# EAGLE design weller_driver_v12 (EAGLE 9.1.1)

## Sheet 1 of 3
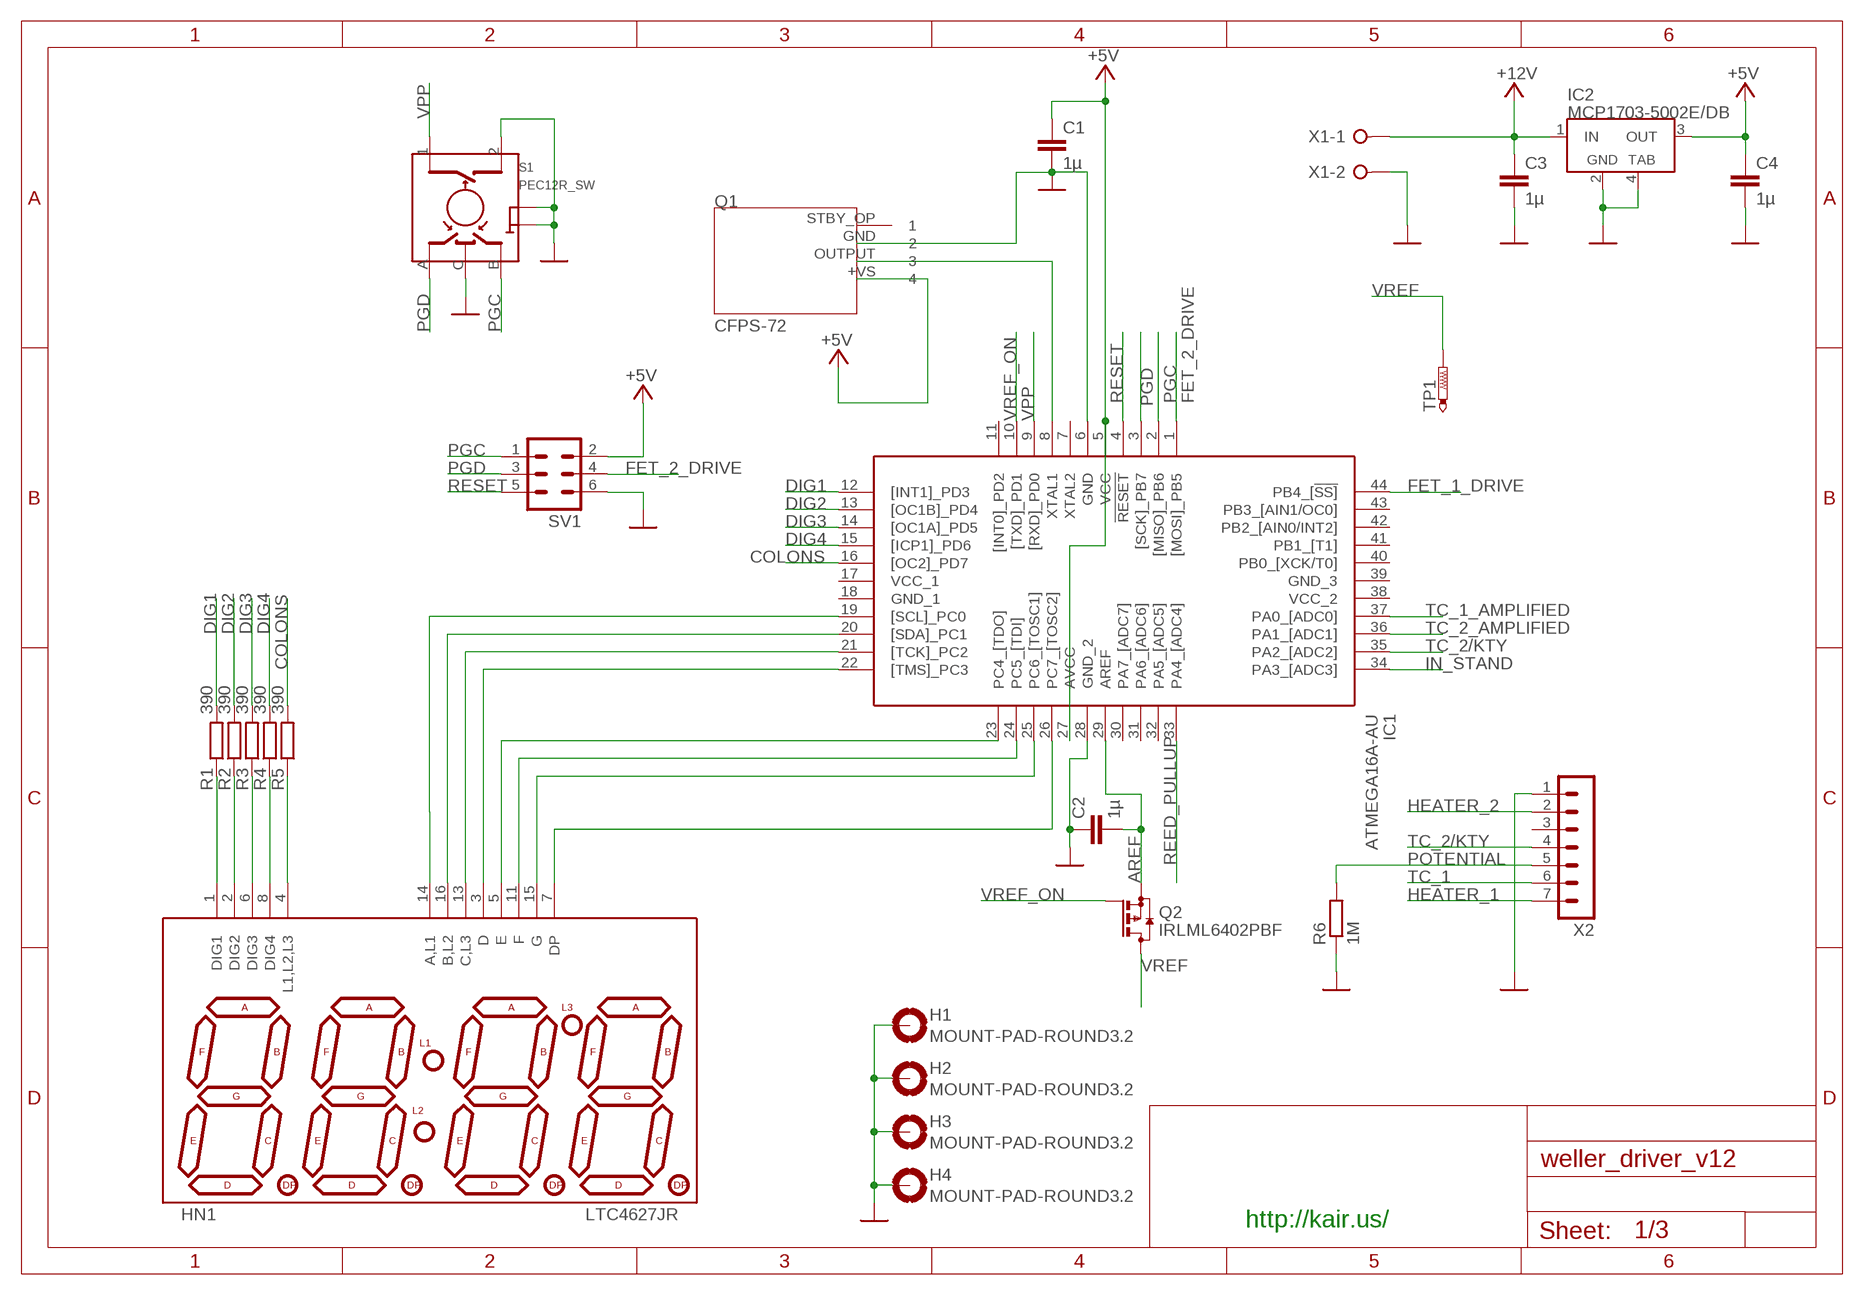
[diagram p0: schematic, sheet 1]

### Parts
C1  1µ  C-EUC0805  [C0805]
C2  1µ  C-EUC0805  [C0805]
C3  1µ  C-EUC0805  [C0805]
C4  1µ  C-EUC0805  [C0805]
H1  MOUNT-PAD-ROUND3.2  [3,2-PAD]
H2  MOUNT-PAD-ROUND3.2  [3,2-PAD]
H3  MOUNT-PAD-ROUND3.2  [3,2-PAD]
H4  MOUNT-PAD-ROUND3.2  [3,2-PAD]
HN1  LTC4627JR  [7-SEGMENT-4DIGIT-YOUNGSUN]
IC1  ATMEGA16A-AU  [ATMEGA16A-AU]
IC2  MCP1703-5002E/DB  VREG_3PIN_FIXED_TAB-SOT223  [SOT223]
Q1  CFPS-72  [CFPS-72]
Q2  IRLML6402PBF  [IRML6402PBF]
R1  390  R-EU_R0805  [R0805]
R2  390  R-EU_R0805  [R0805]
R3  390  R-EU_R0805  [R0805]
R4  390  R-EU_R0805  [R0805]
R5  390  R-EU_R0805  [R0805]
R6  1M  R-EU_R0805  [R0805]
S1  PEC12R_SW  [ALPS_EC12E_SW]
SV1  MA03-2  [MA03-2]
TP1  PTR1PAD1-13  [P1-13]
X1  W237-02P  [W237-132]
X2  MA07-1  [MA07-1]

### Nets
+5V [supply]: C1.1 C4.1 IC1.5(VCC) IC1.27(AVCC) IC2.3(OUT) Q1.+VS SV1.2 ; also sheet 2
+12V [iron_power]: C3.1 IC2.1(IN) X1.1 ; also sheet 2
AREF: C2.2 IC1.29(AREF) Q2.2(S)
COLONS: IC1.16([OC2]_PD7) R5.2
DIG1: IC1.12([INT1]_PD3) R1.2
DIG2: IC1.13([OC1B]_PD4) R2.2
DIG3: IC1.14([OC1A]_PD5) R3.2
DIG4: IC1.15([ICP1]_PD6) R4.2
FET_1_DRIVE: IC1.44(PB4_[!SS]) ; also sheet 2
FET_2_DRIVE: IC1.1([MOSI]_PB5) SV1.4 ; also sheet 2
GND [supply]: C1.2 C2.1 C3.2 C4.2 H1.B3,2(MOUNT) H2.B3,2(MOUNT) H3.B3,2(MOUNT) H4.B3,2(MOUNT) IC1.6(GND) IC1.28(GND_2) IC2.2(GND) IC2.4(GND1) Q1.GND R6.1 S1.2 S1.C S1.GND1(GND) S1.GND2(GND) SV1.6 X1.2 X2.1 ; also sheet 2
HEATER_1 [iron_power]: X2.7 ; also sheet 2
HEATER_2 [iron_power]: X2.2 ; also sheet 2
IN_STAND: IC1.34(PA3_[ADC3]) ; also sheet 2
N$1: HN1.1(DIG1) R1.1
N$2: HN1.2(DIG2) R2.1
N$3: HN1.6(DIG3) R3.1
N$4: HN1.8(DIG4) R4.1
N$7: HN1.5(E) IC1.23(PC4_[TDO])
N$8: IC1.8(XTAL1) Q1.OUTPUT
N$9: HN1.14(A,L1) IC1.19([SCL]_PC0)
N$10: HN1.4(L1,L2,L3) R5.1
N$11: HN1.13(C,L3) IC1.21([TCK]_PC2)
N$13: HN1.16(B,L2) IC1.20([SDA]_PC1)
N$14: HN1.3(D) IC1.22([TMS]_PC3)
N$15: HN1.11(F) IC1.24(PC5_[TDI])
N$16: HN1.15(G) IC1.25(PC6_[TOSC1])
N$17: HN1.7(DP) IC1.26(PC7_[TOSC2])
PGC: IC1.2([MISO]_PB6) S1.B SV1.1
PGD: IC1.3([SCK]_PB7) S1.A SV1.3
POTENTIAL: R6.2 X2.5
REED_PULLUP: IC1.33(PA4_[ADC4]) ; also sheet 2
RESET: IC1.4(!RESET) SV1.5
TC_1: X2.6 ; also sheet 2
TC_1_AMPLIFIED: IC1.37(PA0_[ADC0]) ; also sheet 2
TC_2/KTY: IC1.35(PA2_[ADC2]) X2.4 ; also sheet 2
TC_2_AMPLIFIED: IC1.36(PA1_[ADC1]) ; also sheet 2
VPP: IC1.9([RXD]_PD0) S1.1
VREF: Q2.3(D) TP1.TP ; also sheet 2
VREF_ON: IC1.10([TXD]_PD1) Q2.1(G)
Unconnected: IC1.7(XTAL2) IC1.11([INT0]_PD2) IC1.30(PA7_[ADC7]) IC1.31(PA6_[ADC6]) IC1.32(PA5_[ADC5]) IC1.40(PB0_[XCK/T0]) IC1.41(PB1_[T1]) IC1.42(PB2_[AIN0/INT2]) IC1.43(PB3_[AIN1/OC0]) Q1.STBY_OP X2.3

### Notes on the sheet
- http://kair.us/

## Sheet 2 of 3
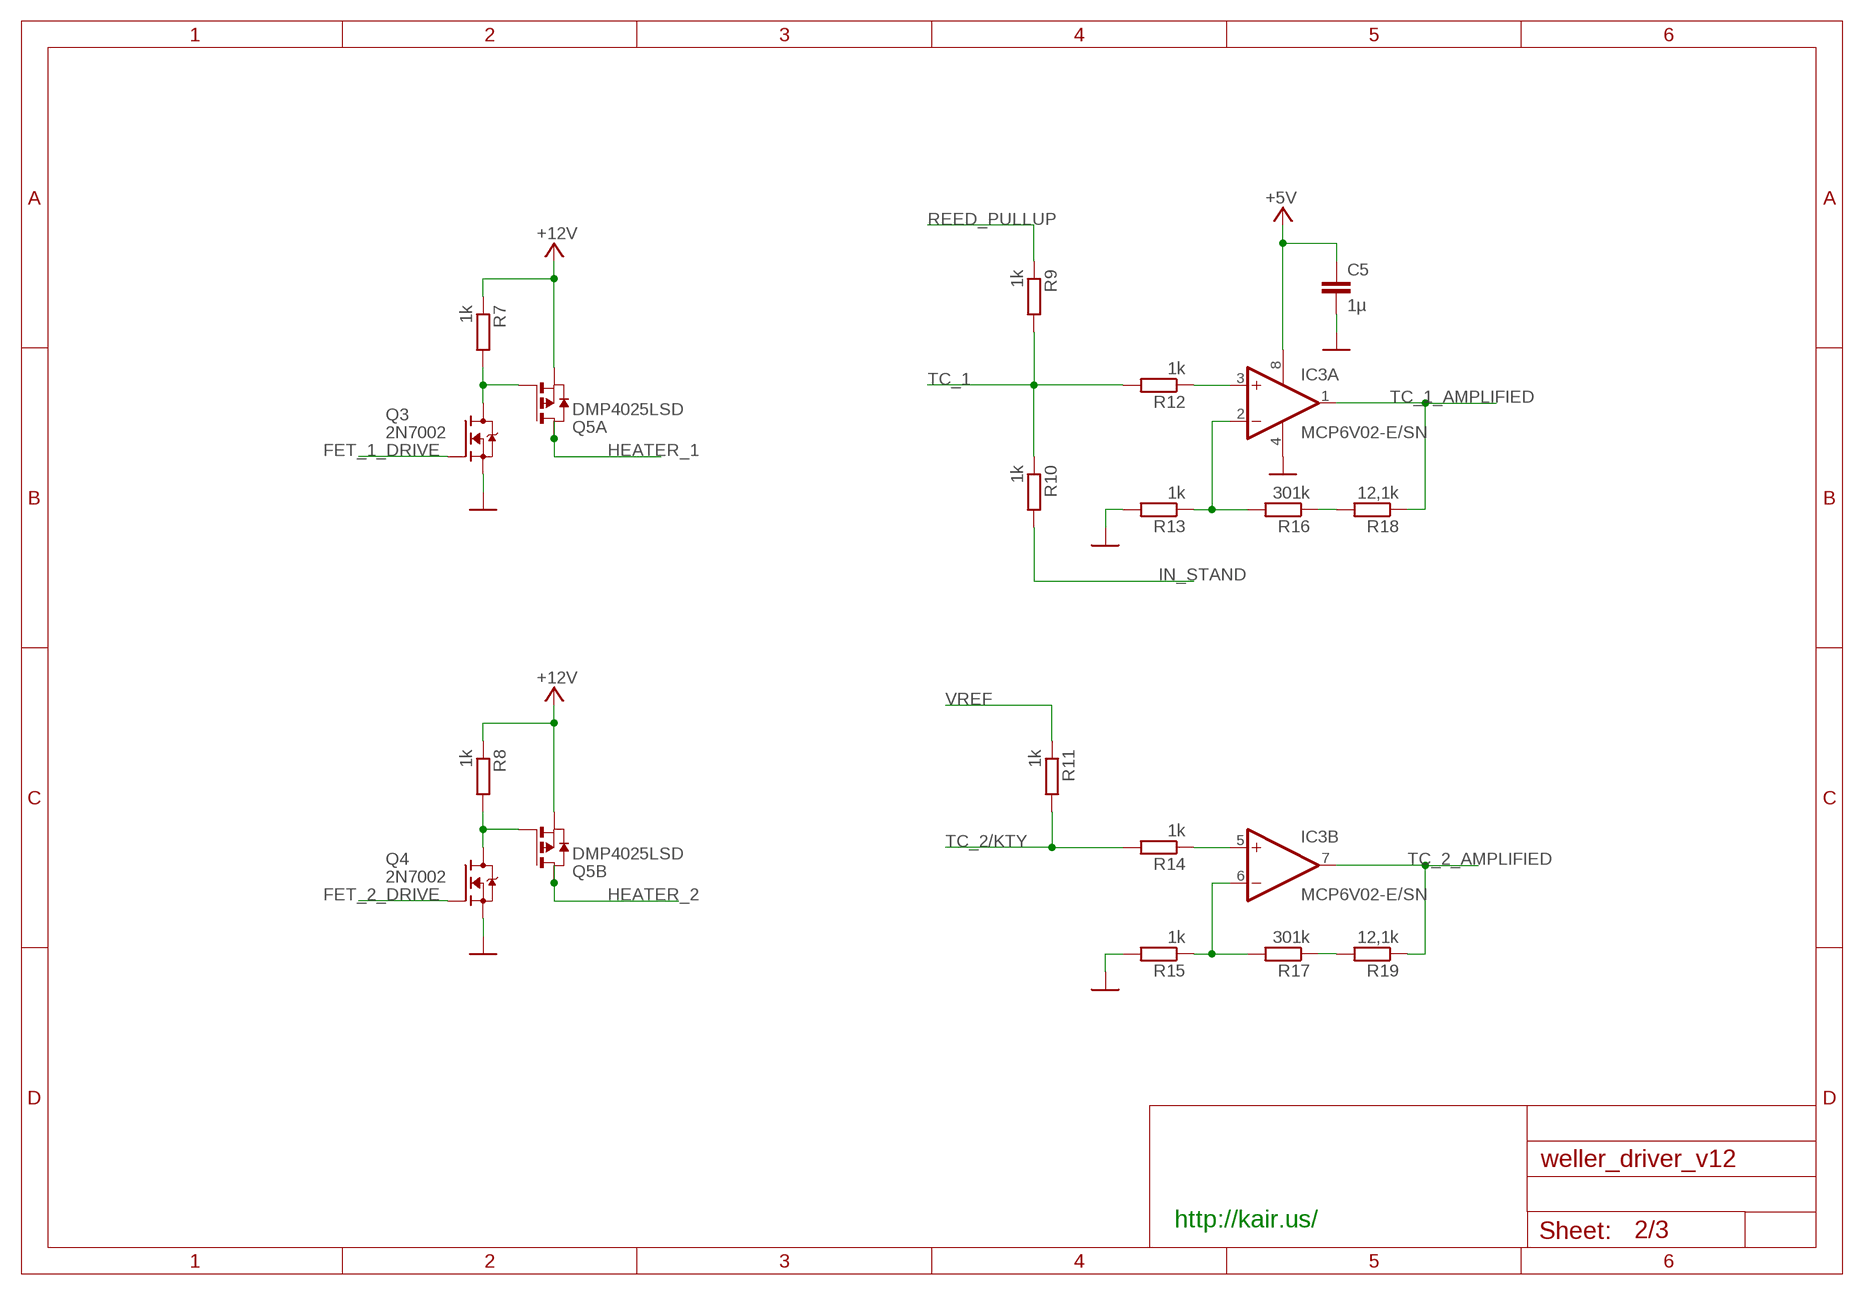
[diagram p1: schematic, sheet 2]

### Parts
C5  1µ  C-EUC0805  [C0805]
IC3  MCP6V02-E/SN  MCP602SN  [SO08]
Q3  2N7002  TRANSISTOR_FET_BS170-SOT-23  [SOT-23]
Q4  2N7002  TRANSISTOR_FET_BS170-SOT-23  [SOT-23]
Q5  DMP4025LSD  PMOS2SO8  [SO08]
R7  1k  R-EU_R0805  [R0805]
R8  1k  R-EU_R0805  [R0805]
R9  1k  R-EU_R0805  [R0805]
R10  1k  R-EU_R0805  [R0805]
R11  1k  R-EU_R0805  [R0805]
R12  1k  R-EU_R0805  [R0805]
R13  1k  R-EU_R0805  [R0805]
R14  1k  R-EU_R0805  [R0805]
R15  1k  R-EU_R0805  [R0805]
R16  301k  R-EU_R0805  [R0805]
R17  301k  R-EU_R0805  [R0805]
R18  12,1k  R-EU_R0805  [R0805]
R19  12,1k  R-EU_R0805  [R0805]

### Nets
+5V [supply]: C5.1 IC3.8(P:V+) ; also sheet 1
+12V [iron_power]: Q5.1(A:S) Q5.3(B:S) R7.1 R8.1 ; also sheet 1
FET_1_DRIVE: Q3.1(G) ; also sheet 1
FET_2_DRIVE: Q4.1(G) ; also sheet 1
GND [supply]: C5.2 IC3.4(P:V-) Q3.2(S) Q4.2(S) R13.2 R15.2 ; also sheet 1
HEATER_1 [iron_power]: Q5.7(A:D) Q5.8(A:D2) ; also sheet 1
HEATER_2 [iron_power]: Q5.5(B:D2) Q5.6(B:D) ; also sheet 1
IN_STAND: R10.2 ; also sheet 1
N$5: R16.1 R18.2
N$6: R17.1 R19.2
N$22: IC3.3(A:+IN) R12.1
N$23: IC3.2(A:-IN) R13.1 R16.2
N$25: IC3.6(B:-IN) R15.1 R17.2
N$27: IC3.5(B:+IN) R14.1
N$28: Q3.3(D) Q5.2(A:G) R7.2
N$42: Q4.3(D) Q5.4(B:G) R8.2
REED_PULLUP: R9.1 ; also sheet 1
TC_1: R9.2 R10.1 R12.2 ; also sheet 1
TC_1_AMPLIFIED: IC3.1(A:OUT) R18.1 ; also sheet 1
TC_2/KTY: R11.2 R14.2 ; also sheet 1
TC_2_AMPLIFIED: IC3.7(B:OUT) R19.1 ; also sheet 1
VREF: R11.1 ; also sheet 1

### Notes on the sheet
- http://kair.us/

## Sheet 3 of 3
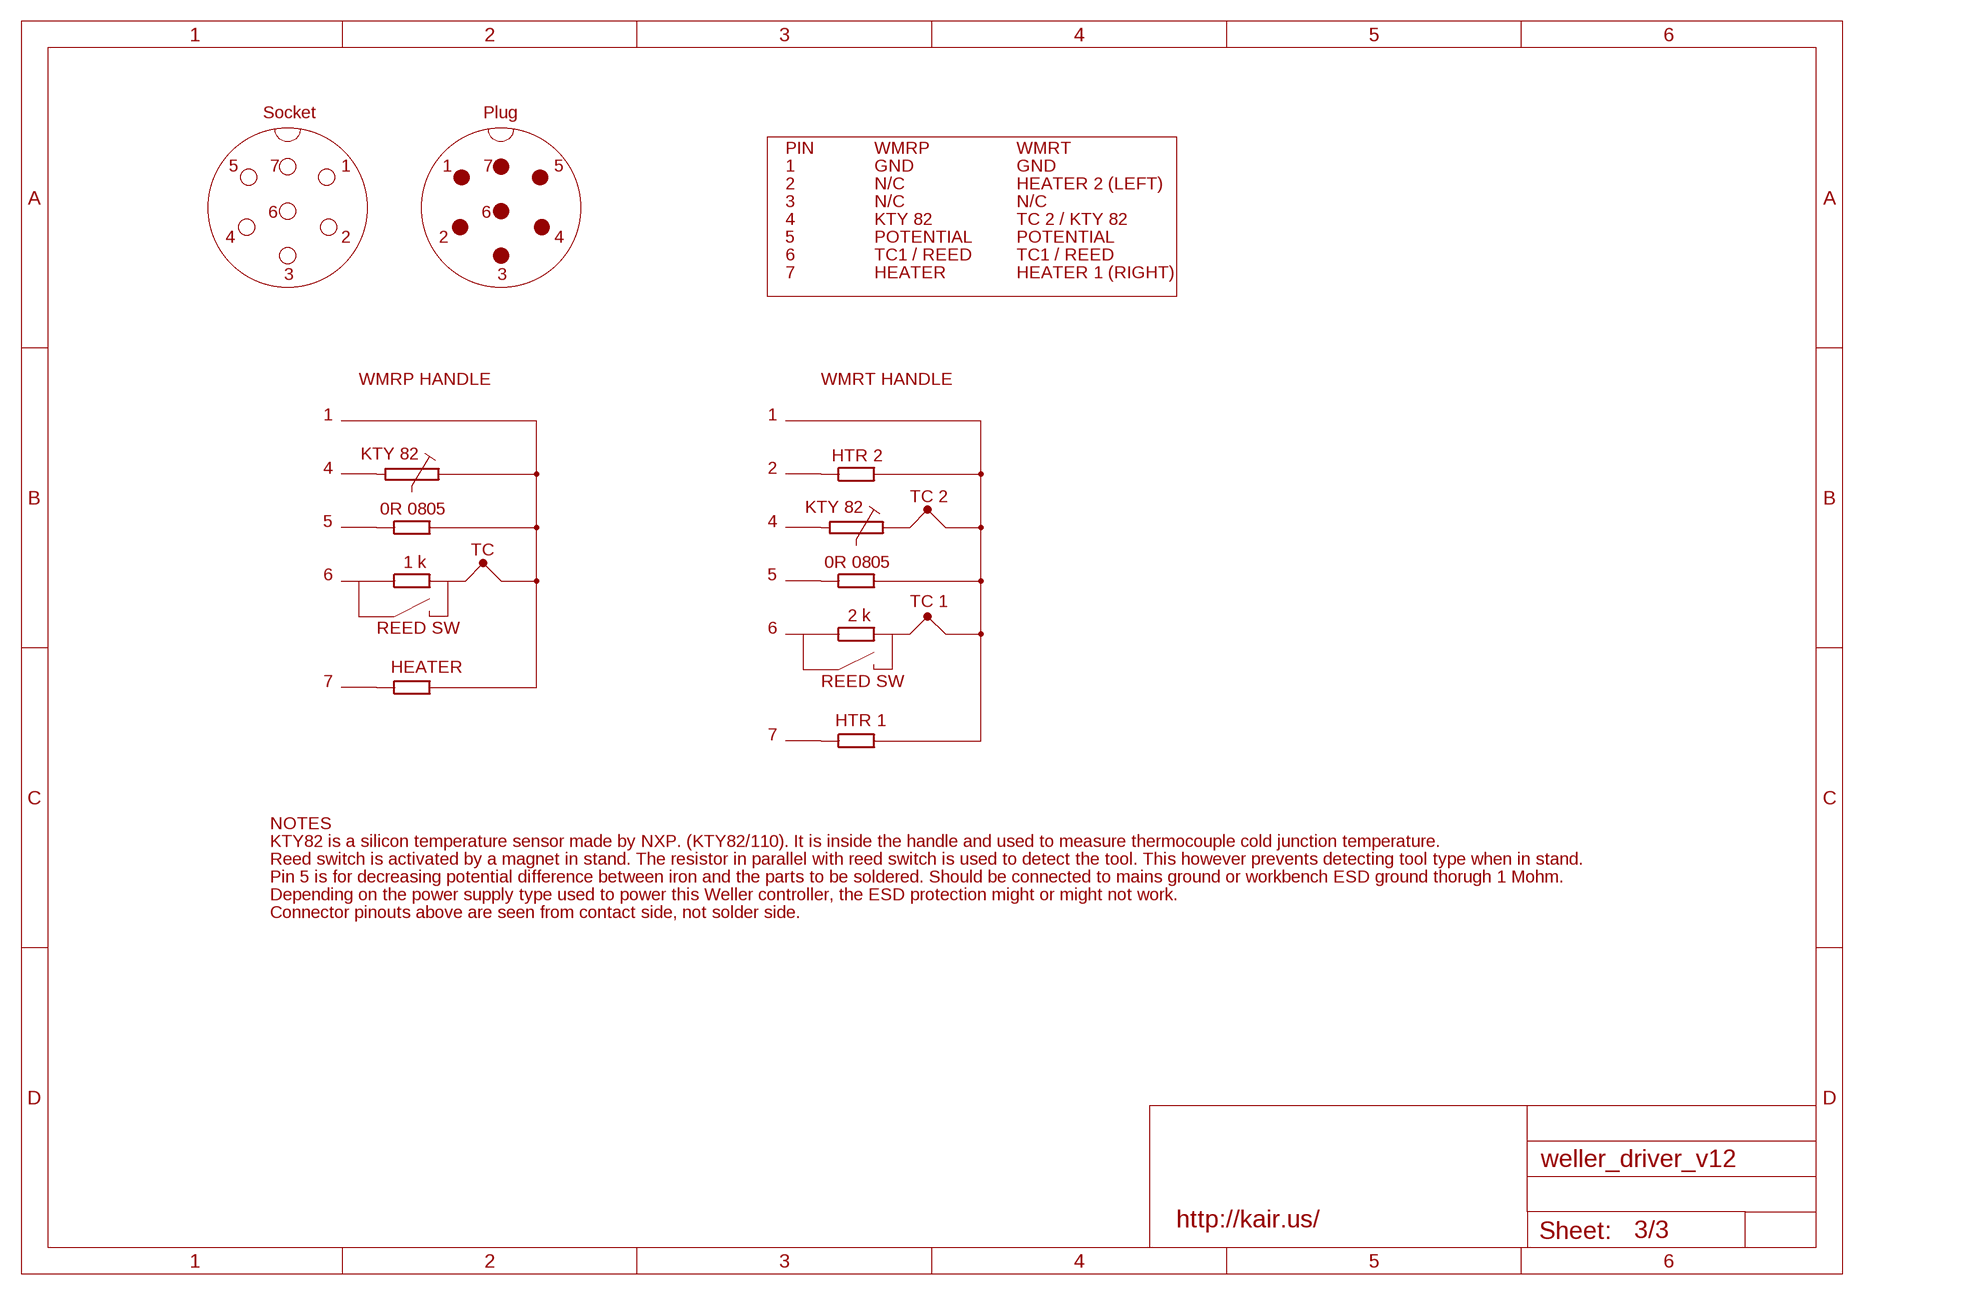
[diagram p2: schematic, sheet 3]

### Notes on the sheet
- Socket | Plug
- PIN | WMRP | WMRT
- 5 | 7 | 1 | 1 | 7 | 5 | 1 | GND | GND
- 2 | N/C | HEATER 2 (LEFT)
- 3 | N/C | N/C
- 6 | 6
- 4 | KTY 82 | TC 2 / KTY 82
- 4 | 2 | 2 | 4 | 5 | POTENTIAL | POTENTIAL
- 6 | TC1 / REED | TC1 / REED
- 3 | 3 | 7 | HEATER | HEATER 1 (RIGHT)
- WMRP HANDLE | WMRT HANDLE
- 1 | 1
- KTY 82 | HTR 2
- 4 | 2
- TC 2
- 0R 0805 | KTY 82
- 5 | 4
- TC
- 1 k | 0R 0805
- 6 | 5
- TC 1
- 2 k
- REED SW | 6
- HEATER
- 7 | REED SW
- HTR 1
- 7
- NOTES
- KTY82 is a silicon temperature sensor made by NXP. (KTY82/110). It is inside the handle and used to measure thermocouple cold junction temperature.
- Reed switch is activated by a magnet in stand. The resistor in parallel with reed switch is used to detect the tool. This however prevents detecting tool type when in stand.
- Pin 5 is for decreasing potential difference between iron and the parts to be soldered. Should be connected to mains ground or workbench ESD ground thorugh 1 Mohm.
- Depending on the power supply type used to power this Weller controller, the ESD protection might or might not work.
- Connector pinouts above are seen from contact side, not solder side.
- http://kair.us/

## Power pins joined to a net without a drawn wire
GND_1: IC1.18(GND_1)
GND_3: IC1.39(GND_3)
VCC_1: IC1.17(VCC_1)
VCC_2: IC1.38(VCC_2)

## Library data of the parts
C1-C5 = dual_atari:C-EU: CAPACITOR, European symbol
H1-H4 = dual_atari:MOUNT-PAD-ROUND: MOUNTING PAD, round
HN1 = omat:LTC4627JR: This is a part for the 4-Digit 7-segment LEDs from Young Sun. Different from the Digikey LEDs, all 16 pins are used. The LONGPADS Variant is used for a test jig, but you may like it because there is more pad to solder to. If you are concerned about routing space, the standard works just fine though.
IC1 = SamacSys_Parts:ATMEGA16A-AU: ATMEGA16A-AU, 8 bit AVR Microcontroller 16MHz 16, 512kB, B Flash, 1kb RAM, I2C SPI 44-Pin TQFP Source: Datasheet; DESCRIPTION: ATMEGA16A-AU, 8 bit AVR Microcontroller 16MHz 16, 512kB, B Flash, 1kb RAM, I2C SPI 44-Pin TQFP; HEIGHT: 1.2mm; MANUFACTURER_NAME: Microchip; MANUFACTURER_PART_NUMBER: ATMEGA16A-AU; MOUSER_PART_NUMBER: 556-ATMEGA16A-AU; MOUSER_PRICE-STOCK: https://www.mouser.com/Search/Refine.aspx?Keyword=556-ATMEGA16A-AU
IC2 = omat:VREG_3PIN_FIXED_TAB
IC3 = omat:MCP602: Single Op Amp 2.7V to 6.0V Single Supply CMOS Source: http://ww1.microchip.com/downloads/en/DeviceDoc/21314g.pdf
Q1 = CFPS-72:CFPS-72
Q2 = IRLML6402PBF:IRLML6402PBF: P-CHANNEL MOS FET
Q3 Q4 = omat:TRANSISTOR_FET_BS170: N-Channel Enhancement Mode Field Effect Transistor
Q5 = omat:PMOS2: DUAL 30V P-CHANNEL ENHANCEMENT MODE MOSFET Source: Data sheet SOP8 Source: Data sheet MSOP8
R1-R19 = dual_atari:R-EU_: RESISTOR, European symbol
S1 = omat:PEC12R_SW
SV1 = con-lstb:MA03-2: PIN HEADER; OC_FARNELL: unknown; OC_NEWARK: unknown
TP1 = testpad:PTR1: TEST PIN
X1 = omat:W237-02P: WAGO SREW CLAMP; OC_FARNELL: unknown; OC_NEWARK: unknown
X2 = omat:MA07-1: PIN HEADER; OC_FARNELL: unknown; OC_NEWARK: unknown

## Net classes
1 supply: width 0.4 mm, drill 0.7 mm, clearance 0.25 mm
2 iron_power: width 1 mm, drill 0.7 mm, clearance 0.25 mm

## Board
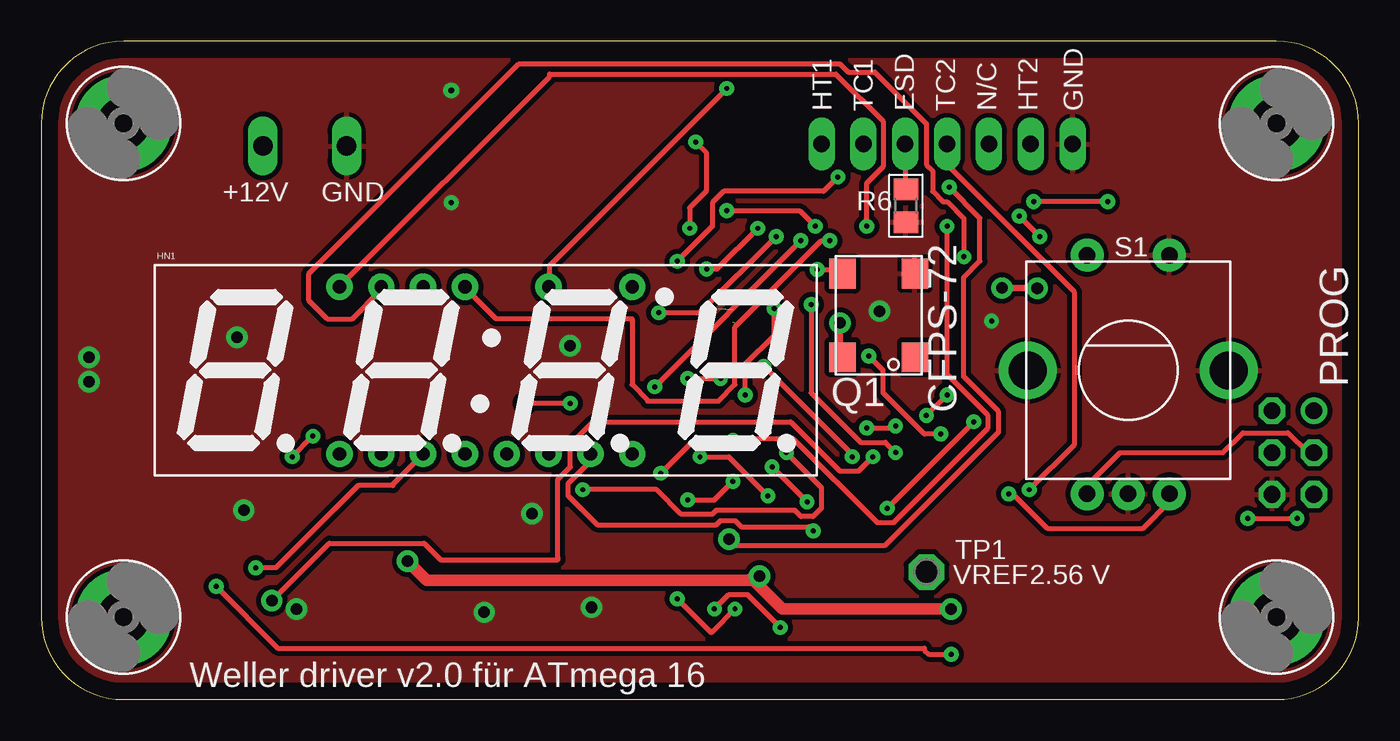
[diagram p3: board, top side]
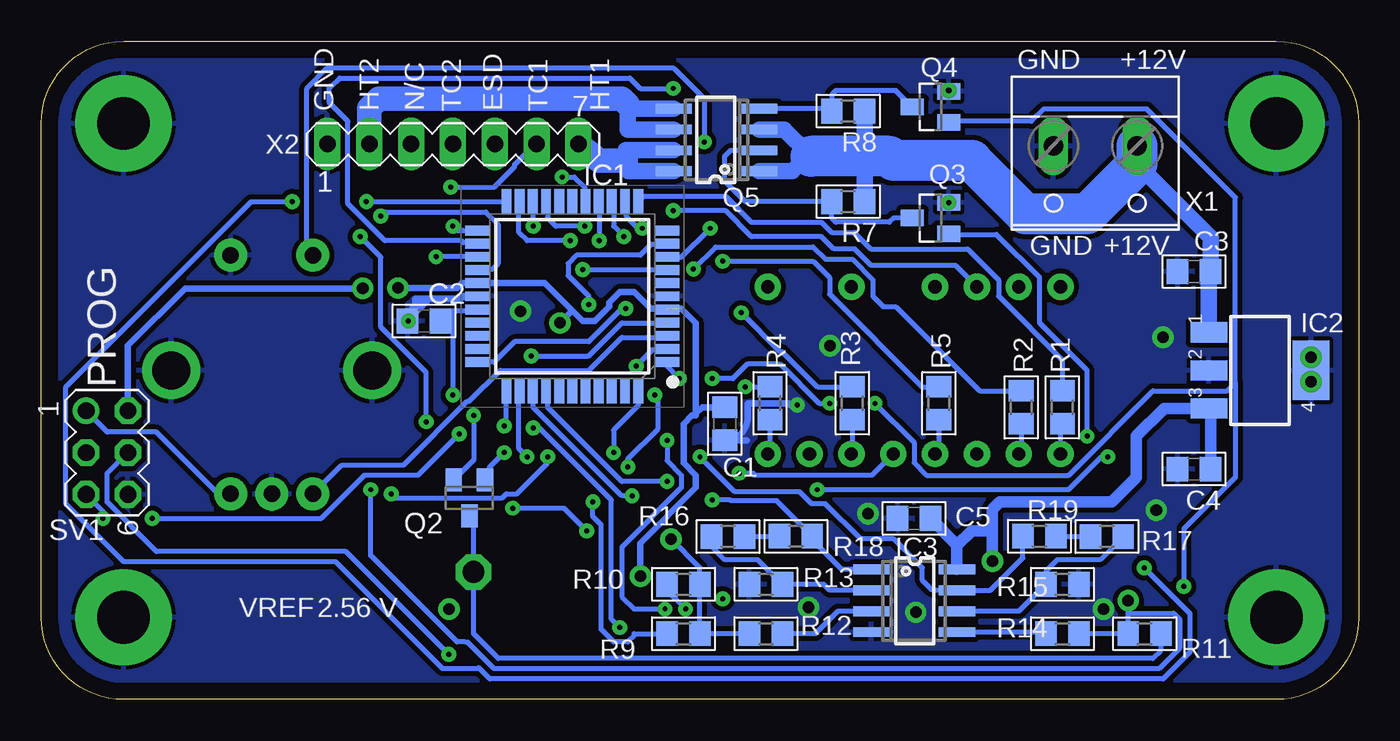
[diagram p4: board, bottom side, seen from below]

Size 80 x 40 mm. Coordinates in mm from the lower left corner, seen from the top.
Outline: 75,0 arc90 80,5 80,35 arc90 75,40 5,40 arc90 0,35 0,5 arc90 5,0 75,0
Copper layers (1*16): Top 0.035mm / dielectric 1.5mm / Bottom 0.035mm
Design rules "default *": minimum track width 0.3mm, minimum drill 0.3mm, track to track 0.25mm, track to pad 0.25mm, pad to pad 0.25mm, via to via 0.25mm, smd to smd 0.25mm, copper to edge 40mil, drill to drill 8mil, minimum pad ring 0.3mm, minimum via ring 0.3mm, stop-mask expansion 4mil, vias tented up to drill 0mil, thermal gap 10mil

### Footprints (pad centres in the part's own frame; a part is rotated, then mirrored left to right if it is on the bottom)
C0805 = smd 1.3 x 1.5: 1 -1,0; 2 1,0
3,2-PAD = drill 3.2 pad 5.842: B3,2 0,0
7-SEGMENT-4DIGIT-YOUNGSUN = drill 0.8 pad 1.6: 1 -8.89,-5.08; 2 -6.35,-5.08; 3 -3.81,-5.08; 4 -1.27,-5.08; 5 1.27,-5.08; 6 3.81,-5.08; 7 6.35,-5.08; 8 8.89,-5.08; 9 8.89,5.08; 11 3.81,5.08; 13 -1.27,5.08; 14 -3.81,5.08; 15 -6.35,5.08; 16 -8.89,5.08
ATMEGA16A-AU = smd 1.5 x 0.6: 1 -5.75,4; 2 -5.75,3.2; 3 -5.75,2.4; 4 -5.75,1.6; 5 -5.75,0.8; 6 -5.75,0; 7 -5.75,-0.8; 8 -5.75,-1.6; 9 -5.75,-2.4; 10 -5.75,-3.2; 11 -5.75,-4; 23 5.75,-4; 24 5.75,-3.2; 25 5.75,-2.4; 26 5.75,-1.6; 27 5.75,-0.8; 28 5.75,0; 29 5.75,0.8; 30 5.75,1.6; 31 5.75,2.4; 32 5.75,3.2; 33 5.75,4 | smd 0.6 x 1.5: 12 -4,-5.75; 13 -3.2,-5.75; 14 -2.4,-5.75; 15 -1.6,-5.75; 16 -0.8,-5.75; 17 0,-5.75; 18 0.8,-5.75; 19 1.6,-5.75; 20 2.4,-5.75; 21 3.2,-5.75; 22 4,-5.75; 34 4,5.75; 35 3.2,5.75; 36 2.4,5.75; 37 1.6,5.75; 38 0.8,5.75; 39 0,5.75; 40 -0.8,5.75; 41 -1.6,5.75; 42 -2.4,5.75; 43 -3.2,5.75; 44 -4,5.75
SOT223 = smd 1.219 x 2.235: 1 -2.311,-3.099; 2 0,-3.099; 3 2.311,-3.099 | smd 3.6 x 2.2: 4 0,3.099
SO08 = smd 0.6 x 2.2: 1 -1.905,-2.6; 2 -0.635,-2.6; 3 0.635,-2.6; 4 1.905,-2.6; 5 1.905,2.6; 6 0.635,2.6; 7 -0.635,2.6; 8 -1.905,2.6
CFPS-72 = smd 1.8 x 1.6: +VS -2.45,2.1; GND 2.63,-2.3; OUTPUT 2.63,2.1; STBY_OP -2.45,-2.3
IRML6402PBF = smd 1 x 1.4: 1 -0.95,-1.1; 2 0.95,-1.1; 3 0,1.1
SOT-23 = smd 1 x 1.4: 1 -0.95,-1.1; 2 0.95,-1.1; 3 0,1.1
R0805 = smd 1.3 x 1.5: 1 -1,0; 2 1,0
ALPS_EC12E_SW = drill 1 pad 2: 1 -2.5,7; 2 2.5,7; A -2.5,-7.5; B 2.5,-7.5; C 0,-7.5 | drill 2.3 pad 3.5: GND1 -6.1,0; GND2 6.1,0
MA03-2 = drill 1.016: 1 -2.54,-1.27 | drill 1.016 octagon: 2 -2.54,1.27; 3 0,-1.27; 4 0,1.27; 5 2.54,-1.27; 6 2.54,1.27
P1-13 = drill 1.321 pad 2.159 octagon: TP 0,0
W237-132 = drill 1.194 long: 1 -2.54,-0.635; 2 2.54,-0.635
MA07-1 = drill 1 long: 1 -7.62,0; 2 -5.08,0; 3 -2.54,0; 4 0,0; 5 2.54,0; 6 5.08,0; 7 7.62,0

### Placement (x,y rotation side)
C1  38.5,16.75 270 bottom
C2  56.75,23 0 bottom
C3  10,26 180 bottom
C4  10,14 180 bottom
C5  27,11 180 bottom
H1  75,35 0 top
H2  5,5 0 top
H3  75,5 0 top
H4  5,35 0 top
HN1  27,20 0 top
IC1  47.75,24.5 180 bottom
IC2  6,20 270 bottom
IC3  27,6 270 bottom
Q1  50.75,23.25 90 top
Q2  54,12.25 180 bottom
Q3  26,29.25 90 bottom
Q4  26,36 90 bottom
Q5  39,34 90 bottom
R1  18,17.75 90 bottom
R2  20.5,17.75 90 bottom
R3  30.75,18 90 bottom
R4  35.75,18 90 bottom
R5  25.5,18 90 bottom
R6  52.5,30 90 top
R7  31,30.25 180 bottom
R8  31,35.75 180 bottom
R9  41,4 0 bottom
R10  41,7 180 bottom
R11  13,4 180 bottom
R12  36,4 180 bottom
R13  36,7 180 bottom
R14  18,4 0 bottom
R15  18,7 0 bottom
R16  38.3,9.9 180 bottom
R17  15.3,9.9 0 bottom
R18  34.18,9.92 180 bottom
R19  19.4,9.92 0 bottom
S1  66,20 0 top
SV1  76,15 270 bottom
TP1  53.75,7.75 0 top
X1  16,33 180 bottom
X2  55,33.75 0 bottom

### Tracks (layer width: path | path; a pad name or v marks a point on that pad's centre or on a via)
+5V  (via drill 0.7)  (1 unrouted)
  Top 0.4: v43.62,7.5 43.5,7.38 43.31,7.19 | v48.5,22.88 48.5,21.12 Q1.+VS | v60.48,24.98 60.45,25 v58.33,25
  Top 0.7: v55.25,5.5 45,5.5 43.31,7.19 43.12,7.38 43,7.25 23.4,7.25 v22.25,8.4
  Bottom 0.4: C1.1 39.88,17.75 40.25,17.38 | v43.62,7.5 43.62,9.5 40.25,12.88 40.25,13.62 41,14.38 41,16.62 41,16.75 40.5,17.25 40.25,17.25 40.25,17.38 | 40.25,17.38 40.25,22.88 41.12,23.75 43,23.75 44,24.75 44.88,24.75 45.5,24.12 45.5,23.88 46.38,23 47.12,23 47.75,23.62 | v48.5,22.88 47.88,23.5 47.75,23.62 | v58.33,25 54.75,25 54.45,25.3 IC1.27 49.42,25.3 47.75,23.62 | SV1.2 74.73,21.5 71.25,24.98 v60.48,24.98
  Bottom 0.5: 9,17.59 IC2.3
  Bottom 0.7: C4.1 9,17.59 | C5.1 24.4,9.4 IC3.8 24.4,9.35 23.5,10.25 22.25,10.25 | IC2.3 11.81,17.69 13.5,16 13.5,13.5 15,12 21.8,12 22.25,11.55 22.25,10.25 | 22.25,10.25 v22.25,8.4
+12V
  Bottom 1: 13.46,32.54 9,28.08 C3.1 9.1,25.9 IC2.1 | R8.1 30,33 R7.1 | Q5.3 34.88,34.63 33.38,33.12 | 33.25,33 33.38,33.12 | Q5.1 34.41,32.09 33.38,33.12
  Bottom 2: 28.25,32.75 28.5,33
  Bottom 2.5: X1.1 13.46,32.54 16.5,29.5 20.25,29.5 23.5,32.75 28.25,32.75 | 28.5,33 30,33 33.25,33
AREF  (via drill 0.3)
  Top 0.3: v55,18.5 v53.75,17.25
  Bottom 0.3: 55.06,23.56 55.62,23 C2.2 | 55.06,23.56 55,23.62 53.5,23.62 IC1.29 | v55,18.5 55,23.5 55.06,23.56 | v53.75,17.25 53.75,14.55 Q2.2
COLONS  (via drill 0.3)
  Top 0.3: v48.38,31.75 47.5,30.88 41.45,30.88 40.75,30.18 40.75,28.75 v38.62,26.62
  Bottom 0.3: v48.38,31.75 47.62,31.75 47,31.12 47,30.38 IC1.16 | v38.62,26.62 33.12,26.62 32.12,25.62 32.12,24.62 26.5,19 25.62,19 R5.2
DIG1
  Bottom 0.3: R1.2 18,20.62 21.88,24.5 21.88,25.5 23.75,27.38 29.62,27.38 30.62,28.38 32,28.38 32.62,29 36.88,29 38.45,30.57 43.42,30.57 IC1.12
DIG2  (via drill 0.3)
  Top 0.3: v40.4,26.15 41.02,26.15 v43.5,28.62
  Bottom 0.3: R2.2 23,18.75 28.12,23.88 28.88,23.88 29.5,24.5 29.5,25.5 30.75,26.75 32.38,26.75 33.12,27.5 39.05,27.5 v40.4,26.15 | v43.5,28.62 43.75,28.62 44.5,29.38 44.5,30.12 IC1.13
DIG3  (via drill 0.3)
  Top 0.3: v44.62,28.12 40,23.5 v37.5,23.5
  Bottom 0.3: R3.2 32.88,19 35,21.12 35.12,21.12 v37.5,23.5 | v44.62,28.12 45.25,28.75 45.25,30.15 IC1.14
DIG4  (via drill 0.3)
  Top 0.3: v46.12,27.88 v37.25,19
  Bottom 0.3: v37.25,19 R4.2 | IC1.15 46.12,30.23 v46.12,27.88
FET_1_DRIVE  (via drill 0.3)
  Top 0.3: v15.25,14.75 v16.5,16 | v32.88,12.75 37.38,12.75 38.88,11.25 40.75,11.25 41,11.5 45.75,11.5 46.12,11.12 46.88,11.12 47.38,11.62 47.38,12.88 v45.25,15
  Bottom 0.3: v16.5,16 16.5,20 19.38,22.88 19.38,25.62 22,28.25 24.85,28.25 Q3.1 | v15.25,14.75 15.62,14.75 17.62,12.75 v32.88,12.75 | v45.25,15 45.25,16.38 43.75,17.88 IC1.44
FET_2_DRIVE  (via drill 0.3)
  Top 0.3: v32.12,18 v29.38,18 | v10.62,6.88 14.38,3.12 53.62,3.12 53.62,3 53.88,2.75 v55.25,2.75 | v39.25,19.5 v41.25,19.5
  Bottom 0.3: 7.5,19.25 7.5,30.5 12.88,35.88 19.12,35.88 19.88,35.12 24.88,35.12 Q4.1 | 7.5,19.25 8,18.75 12.5,18.75 17.62,13.62 26.25,13.62 27,14.38 27,15.62 v29.38,18 | v32.12,18 32.75,18 35.12,20.38 35.25,20.38 37.12,20.38 38,19.5 v39.25,19.5 | v10.62,6.88 10.62,10.38 7.5,13.5 7.5,19.12 7.5,19.25 | IC1.1 42,20.25 v41.25,19.5 | v55.25,2.75 61.5,9 73,9 76,12 76,13.73 SV1.4
GND  (via drill 0.3, 0.35, 0.7)
  Bottom 0.4: 37.15,15.75 C1.2 arc-90 37.1,17.15 37.1,18 34.65,18 arc90 34.55,17.9 | 57.35,23.4 C2.1 | 54.33,24.5 IC1.28 53.55,24.45 54.38,24.45 54.33,24.5 | 56.44,24.35 57.3,24.35 57.3,23.45 C2.1 | 56.4,24.35 56.44,24.35 | 56.44,24.35 56.59,24.2 | 56.4,24.35 54.54,24.35 54.33,24.5 | C2.1 56.85,23.9 56.85,23.94 56.59,24.2 | 56.59,24.2 56.55,24.2 56.4,24.35 | C2.1 57.75,23.04 arc90 56.59,24.2
  other vias: 2.9,20.8 2.9,19.3 12.3,11.5 15.5,5.5 26.9,5.3 29.8,11.3 11.9,22 57.7,23 50.9,23.6 24.9,30.2 24.9,37 33.4,5.6 34.1,17.9 32.1,21.5
  pour Top (isolate 0.3): 5,0 75,0 arc90 80,5 80,35 arc90 75,40 5,40 arc90 0,35 0,5 arc90
  pour Bottom (isolate 0.3): 5,0 75,0 arc90 80,5 80,35 arc90 75,40 5,40 arc90 0,35 0,5 arc90
HEATER_1
  Bottom 1: Q5.7 44.5,33.37 44.5,32.75 44.5,32.25 44.34,32.09 Q5.8
  Bottom 1.5: X2.7 46.13,32.75 44.5,32.75
HEATER_2
  Bottom 1: Q5.6 44.38,34.63 44.38,35.75 | 44.38,35.75 44.38,36.13 | Q5.5 44.23,35.91 44.38,35.75
  Bottom 1.5: X2.2 60.08,35.92 59.5,36.5 44.75,36.5 44.38,36.13
IN_STAND  (via drill 0.3)
  Top 0.3: v51.88,16.62 51.75,16.5 v50.12,16.5 | v44.88,4.38 42.88,6.38 41.75,6.38 v40.88,5.5
  Bottom 0.3: IC1.34 51.75,16.75 v51.88,16.62 | v50.12,16.5 49.75,16.5 45.38,12.12 45.38,4.88 v44.88,4.38 | v40.88,5.5 42.25,6.88 R10.2
N$1
  Bottom 0.3: HN1.1 18.11,16.64 R1.1
N$2
  Bottom 0.3: R2.1 20.5,15.07 HN1.2
N$3
  Bottom 0.3: R3.1 30.75,14.98 HN1.6
N$4
  Bottom 0.3: R4.1 35.75,15.06 HN1.8
N$5
  Bottom 0.3: R16.1 35.21,9.9 R18.2
N$6
  Bottom 0.3: R19.2 18.38,9.9 R17.1
N$7  (via drill 0.3)
  Top 0.3: v38.62,6.12 40.69,4.06 40.75,4.12 v42.12,5.5 | v55,28.75 55,24.3 55,19.75 57.5,17.25 57.5,16.5 51.75,10.75 50.75,10.75 45.62,15.88 42,15.88 | 42,15.88 39.75,15.88 v37.62,13.75 | v42,15.75 42,15.88
  Bottom 0.3: IC1.23 54.38,28.5 54.5,28.5 54.75,28.5 v55,28.75 | v37.62,13.75 36.75,13.75 36.75,13.62 29.57,13.62 HN1.5 | v42.12,5.5 44,5.5 44.75,6.25 44.75,9.25 41.12,12.88 41.12,13.62 42,14.5 v42,15.75
N$8  (via drill 0.3)
  Top 0.3: v47.12,26.12 48.41,26.12 Q1.OUTPUT
  Bottom 0.3: v47.12,26.12 42.12,26.12 IC1.8
N$9  (via drill 0.3)
  Top 0.3: v47,28.75 46.05,29.7 v41.62,29.7
  Bottom 0.3: v47,28.75 48.75,28.75 49.25,29.25 49.25,30.15 IC1.19 | v41.62,29.7 38.45,29.7 36.88,28.12 32.62,28.12 31.88,27.38 30.6,27.38 29.6,26.38 24.48,26.38 HN1.14
N$10
  Bottom 0.3: R5.1 25.5,15.15 HN1.4
N$11  (via drill 0.3)
  Top 0.3: v47.88,27.88 47.38,27.88 42.12,22.62 42.12,19.12 41.12,18.12 36.8,18.12 36.8,18.2 35.88,19.12 35.88,23.12 35.75,23.12 27.62,23.12 25.73,25.02 HN1.13
  Bottom 0.3: v47.88,27.88 50.5,27.88 51,28.38 51,30.12 IC1.21
N$13  (via drill 0.3)
  Top 0.3: v50.12,28.75 50.12,31.38 51.12,32.38 51.12,35.12 48.25,38 30.88,38 30.88,37.84 HN1.16
  Bottom 0.3: v50.12,28.75 50.12,30.12 IC1.20
N$14  (via drill 0.3)
  Top 0.3: v13.03,8 14.25,8 19.25,13 21.38,13 21.38,13.11 HN1.3 | v64.75,30.25 v60.25,30.25
  Bottom 0.3: IC1.22 54,30.25 54.12,30.25 v60.25,30.25 | v13.03,8 10.25,5.22 10.25,2.88 11.88,1.25 52.75,1.25 53.44,1.94 53.5,1.88 55.62,1.88 62.12,8.38 75,8.38 78.5,11.88 78.5,19 67.25,30.25 v64.75,30.25
N$15  (via drill 0.3)
  Top 0.3: v41.62,37.12 30.88,26.38 30.88,25.14 arc-90 HN1.11
  Bottom 0.3: IC1.24 53.62,27.75 54.38,27.75 54.5,27.88 59.12,27.88 61.38,30.12 61.38,35.12 62.5,36.25 62.5,37.12 62.5,37.25 62.38,37.25 61.88,37.75 44.25,37.75 43.62,37.12 v41.62,37.12
N$16  (via drill 0.3)
  Top 0.3: v56.02,26.9 56.02,29.23 55,30.25 54.75,30.25 54.12,30.88 54.12,32.12 53.75,32.5 53.75,35 50.62,38.12 49,38.12 48.5,38.62 29,38.62 16.25,25.88 16.25,24.25 17.38,23.12 18.88,23.12 20.65,24.9 HN1.15
  Bottom 0.3: IC1.25 v56.02,26.9
N$17  (via drill 0.3)
  Top 0.3: v60.62,28.12 v59.38,29.38 | v51.38,11.62 v56.62,16.88 | v46.88,10.25 46.62,10.5 42.5,10.5 42.12,10.88 41.25,10.88 41,10.62 33.75,10.62 32,12.38 32,13.12 33.35,14.47 HN1.7
  Bottom 0.3: v59.38,29.38 59.12,29.62 53,29.62 52.25,28.88 52.25,26.5 52.62,26.12 53.38,26.12 IC1.26 | v60.62,28.12 59.38,26.88 59.38,22.62 56.62,19.88 v56.62,16.88 | v51.38,11.62 48.25,11.62 v46.88,10.25
N$22
  Bottom 0.3: IC3.3 31.64,5.37 33,4 R12.1
N$23
  Bottom 0.3: IC3.2 32.13,6.63 32.5,7 R13.1 36.5,8.5 38.5,8.5 39.3,9.3 R16.2
N$25
  Bottom 0.3: IC3.6 20.64,5.37 R15.1 19,7.8 18.3,8.5 15.7,8.5 R17.2
N$27
  Bottom 0.3: 19.09,4.09 IC3.5
  Bottom 0.5: R14.1 19.09,4.09
N$28
  Bottom 0.3: Q5.2 38.13,33.37 38.5,33 38.5,31.5 37.25,30.25 R7.2 32,29.25 31.75,29 28.5,29 28.25,29.25 Q3.3
N$42
  Bottom 0.3: Q5.4 32.09,35.91 R8.2 32,36.75 31.75,37 28.1,37 Q4.3
PGC  (via drill 0.3)
  Top 0.3: v43.88,20.25 49.25,14.88 v49.25,14.75 | v58.75,12.5 59,12.5 61.12,10.38 66.88,10.38 68.5,12 S1.B
  Bottom 0.3: v43.88,20.25 42.88,21.25 42.12,21.25 IC1.2 | v49.25,14.75 49.25,14.38 51.12,12.5 51.75,12.5 52,12.25 58.5,12.25 v58.75,12.5 | SV1.1 75.98,16.25 73,16.25 69.25,12.5 | 69.25,12.5 S1.B 69.25,12.5
PGD
  Top 0.3: S1.A 63.5,13 65.5,15 71.75,15 72.96,16.21 75.69,16.21 76.89,15 SV1.3
  Bottom 0.3: S1.A 61.75,14.25 58,14.25 54.12,18.12 54,18.12 52.12,20 46.75,20 44.75,22 42.12,22 IC1.3
POTENTIAL
  Top 0.3: X2.5 52.46,31.04 R6.2
REED_PULLUP  (via drill 0.3)
  Top 0.3: v44.5,23.75 44.5,22.12 42.75,20.38 v42.75,18.5 | v46.5,12 v44.38,14.12
  Bottom 0.3: R9.1 44,4 44,3.88 44.38,3.5 45.25,3.5 46,4.25 46,10.62 46.5,11.12 v46.5,12 | IC1.33 52.5,20.5 51.25,21.75 46.75,21.75 44.75,23.75 v44.5,23.75 | v44.38,14.12 44.38,14.62 42.55,16.45 42.55,18.3 v42.75,18.5
RESET  (via drill 0.3)  (1 unrouted)
  Top 0.3: v50.25,20.88 51.12,20 51.12,18.62 53.62,16.12 v54.62,16.12 | v73.25,11 v76.25,11
  Bottom 0.3: 42.12,22.88 44.75,22.88 46.75,20.88 v50.25,20.88 | v73.25,11 63,11 60.38,13.62 57.12,13.62 v54.62,16.12 | SV1.5 76.25,11.44 v76.25,11
TC_1  (via drill 0.3, 0.7)
  Top 0.3: v55.12,31.12 57,29.25 57,26.62 56,25.62 56,19.62 58.12,17.5 58.12,16.25 51.25,9.38 42.12,9.38 v41.75,9.75
  Bottom 0.3: R12.2 R9.2 R10.1 40,8 v41.75,9.75 | v55.12,31.12 52.5,31.12 51.25,32.38 51.25,32.5 50,33.75 X2.6
TC_1_AMPLIFIED  (via drill 0.3)
  Top 0.3: v42,13.25 40.88,12.12 v39.25,12.12
  Bottom 0.3: IC3.1 31.41,7.91 33.5,10 33.26,10 R18.1 35.33,12.07 38.1,12.07 38.15,12.12 v39.25,12.12 | v42,13.25 44.75,13.25 49.25,17.75 49.25,18.62 IC1.37
TC_2/KTY  (via drill 0.3, 0.7)
  Top 0.3: v14,6 17.5,9.5 23.25,9.5 24.25,8.5 31.38,8.5 31.38,8.62 31.38,13.38 32.12,14.12 32.12,15.5 33.5,16.88 45.5,16.88 48.5,13.88 49.62,13.88 v50.5,14.75 | X2.4 55,32.5 62.75,24.75 62.75,15.5 v60,12.75
  Bottom 0.3: R14.2 R11.2 14,5.25 | 14,5.25 v14,6 | 14,5.25 13.88,5.25 11.25,5.25 10.88,4.88 10.88,3.12 12.12,1.88 52.5,1.88 54.12,3.5 54.25,3.5 54.75,3.5 60,8.75 v60,12.75 | v50.5,14.75 51,15.25 51,18.62 IC1.35
TC_2_AMPLIFIED  (via drill 0.3)
  Top 0.3: v44.12,12.38 41.75,14.75 v40,14.75
  Bottom 0.3: v40,14.75 37.88,12.62 33.95,12.62 33.23,11.9 32.38,11.9 30.23,9.75 28.25,9.75 26.5,8 26.5,7.25 25.89,6.63 IC3.7 22.36,6.63 20.4,8.6 R19.1 | v44.12,12.38 44.75,12.38 50.12,17.75 50.12,18.62 IC1.36
VPP  (via drill 0.3)
  Top 0.3: v39.38,28.62 39.38,29.88 40.38,30.88 40.38,33.25 v39.75,33.88
  Bottom 0.3: v39.38,28.62 41.12,26.88 41.98,26.88 IC1.9 | v39.75,33.88 39.75,36.5 41.62,38.38 62.62,38.38 63.88,37.12 63.88,27.38 S1.1
VREF
  Bottom 0.3: R11.1 12,3 12.5,2.5 52.25,2.5 53.75,4 TP1.TP 53.75,10.9 Q2.3
VREF_ON  (via drill 0.3)
  Top 0.3: v51.88,15 51.25,15.62 49.75,15.62 46.75,18.62 v46.75,24
  Bottom 0.3: v46.75,24 46.75,24.5 48,25.75 48,26.5 47.5,27 43.62,27 43,27.62 42.12,27.62 IC1.10 | Q2.1 52.81,14.06 v51.88,15

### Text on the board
tPlace: HT1 | TC1 | ESD | TC2 | N/C | HT2 | GND | +12V | GND | PROG | VREF | 2.56 V | Weller driver v2.0 für ATmega 16
bPlace: +12V | GND | HT1 | TC1 | ESD | TC2 | N/C | HT2 | GND | +12V | GND | 2.56 V | VREF
bNames: PROG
